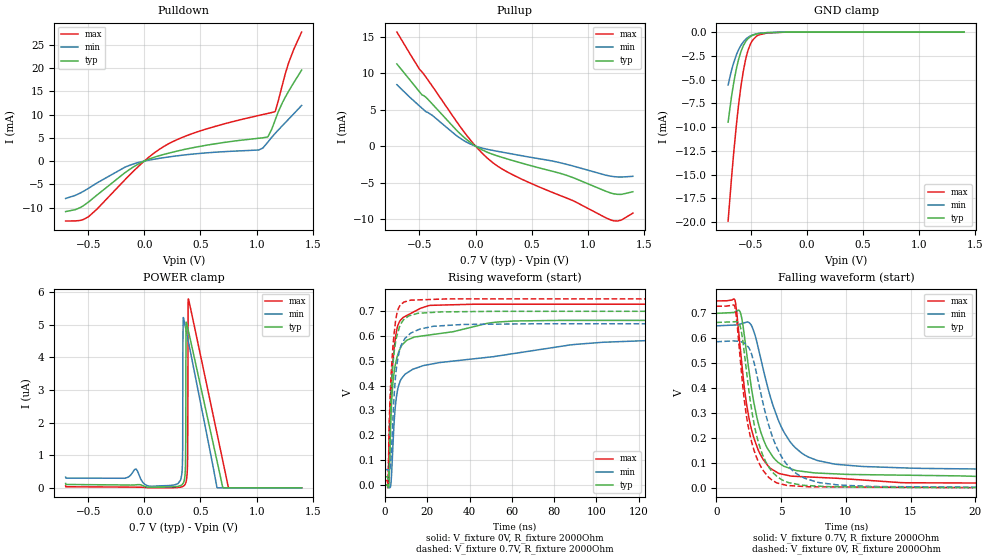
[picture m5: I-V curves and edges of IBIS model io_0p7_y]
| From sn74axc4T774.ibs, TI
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|   io_0p7_y Model
[Model]   io_0p7_y
Model_type   I/O
Polarity   Non-Inverting
Enable   Active-Low
Vinl = 0.21
Vinh = 0.49
Vmeas = 0.35
Vref = 0
Cref = 2pF
Rref = 100000
|   typ   min   max
C_comp   1.852pF   1.651pF   2.136pF
[Model spec]
|subparameter
Vinl   0.21   0.195   0.225
Vinh   0.49   0.455   0.525
| Where Nom  PVT is Nominal Process, 0.7V, 27C
|   Fast PVT is Strong Process,  0.75V, -40C
|   Slow PVT is Weak Process,   0.65V, 130C
[Voltage Range]   0.7   0.65   0.75
|Junction Temperature
[Temperature Range]   27   130   -40
[Pullup Reference]   0.7   0.65   0.75
[Pulldown Reference]   -0   0   0
[Power Clamp Reference]   0.7   0.65   0.75
[GND Clamp Reference]   0   0   0
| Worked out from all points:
|   slope of the pulldown table from 0 to 0.105 V, typ, clamps not added: 111 ohm
|   slope of the pullup table from 0 to 0.105 V, typ, clamps not added: 124 ohm
|   GND clamp passes 1 mA (typ) near -0.54 V on its own axis
|   falling waveform, V_fixture 0.7V, R_fixture 2000Ohm: 20-80 % time 1.59ns typ, 2.42ns min, 1.38ns max; typ from 0.7 V to 0.033 V
|   rising waveform, V_fixture 0V, R_fixture 2000Ohm: 20-80 % time 3.92ns typ, 10.6ns min, 2.96ns max; typ from 0 V to 0.663 V
|   rising waveform, V_fixture 0.7V, R_fixture 2000Ohm: 20-80 % time 2.57ns typ, 3.32ns min, 2.42ns max; typ from 0.033 V to 0.7 V
|   falling waveform, V_fixture 0V, R_fixture 2000Ohm: 20-80 % time 1.39ns typ, 2.07ns min, 1.21ns max; typ from 0.663 V to 0 V
[Pulldown]
|   Voltage   I(typ)   I(min)   I(max)
-700mV    -10.84mA   -8.039mA   -12.88mA
-613.9mV  -10.44mA   -7.366mA   -12.86mA
-496.3mV  -8.79mA    -5.848mA   -11.95mA
-86.8mV   -1.114mA   -543.1uA   -1.949mA
74.9mV    709.2uA    349.2uA    1.494mA
230.3mV   1.783mA    928.3uA    3.893mA
528.5mV   3.299mA    1.714mA    6.718mA
1.018V    4.901mA    2.379mA    9.794mA
1.098V    5.18mA     4.003mA    10.23mA
1.163V    8.678mA    5.897mA    10.62mA
1.282V    14.92mA    8.955mA    20.95mA
1.4V      19.54mA    11.95mA    27.72mA
[GND Clamp]
|   Voltage   I(typ)   I(min)   I(max)
-700mV    -9.473mA   -5.569mA   -19.87mA
-674.8mV  -7.198mA   -4.264mA   -16.07mA
-649.6mV  -5.285mA   -3.192mA   -12.61mA
-622.3mV  -3.629mA   -2.276mA   -9.304mA
-584.5mV  -2.013mA   -1.371mA   -5.599mA
-544.6mV  -1.015mA   -772.1uA   -2.899mA
-521.5mV  -677.6uA   -547uA     -1.878mA
-481.6mV  -348uA     -300.8uA   -843.7uA
-443.8mV  -200.2uA   -174.6uA   -401uA
-351.4mV  -69.33uA   -55.44uA   -97.88uA
-175mV    -6.308uA   -6.304uA   -6.326uA
1.4V      0A         0A         0A
[Pullup]
|   Voltage   I(typ)   I(min)   I(max)
-700mV    11.25mA    8.412mA    15.63mA
-500.5mV  7.467mA    5.518mA    10.57mA
-424.9mV  6.427mA    4.607mA    9.085mA
-145.6mV  1.818mA    1.166mA    2.856mA
-7mV      68.33uA    37.43uA    122.1uA
148.4mV   -1.105mA   -579uA     -2.212mA
263.9mV   -1.677mA   -908.2uA   -3.386mA
410.9mV   -2.34mA    -1.323mA   -4.536mA
793.1mV   -3.921mA   -2.435mA   -7.018mA
1.203V    -6.426mA   -4.123mA   -10.12mA
1.291V    -6.618mA   -4.243mA   -10.17mA
1.4V      -6.259mA   -4.143mA   -9.188mA
[POWER Clamp]
|   Voltage   I(typ)   I(min)   I(max)
-700mV    133.1nA    328.5nA    61.75nA
301.7mV   46.57nA    137.1nA    11.38nA
337.4mV   102.3nA    571.4nA    34.33nA
341.6mV   118.7nA    1.205uA    40.17nA
345.8mV   140.3nA    5.138uA    47.42nA
362.6mV   405.2nA    4.989uA    104.1nA
368.9mV   1.505uA    4.883uA    151.5nA
371mV     4.89uA     4.848uA    174.5nA
385.7mV   4.915uA    4.597uA    910.4nA
392mV     4.819uA    4.489uA    5.793uA
751.1mV   0A         0A         0A
1.4V      0A         0A         0A
[Ramp]
R_load = 2000
|   typ   min   max
dV/dt_r   0.398078/3.88391e-09   0.351677/1.04111e-08   0.437151/2.93764e-09
dV/dt_f   0.400332/1.59305e-09   0.352882/2.41142e-09   0.439509/1.3705e-09
[Falling Waveform]
V_fixture = 0.7V
V_fixture_min = 0.65V
V_fixture_max = 0.75V
R_fixture = 2000Ohm
C_fixture = 0F
|   Time   V(typ)   V(min)   V(max)
0s        700mV      650mV      750mV
1.435ns   705.8mV    653.3mV    753.6mV
1.852ns   704.2mV    657.3mV    560.5mV
2.701ns   404.1mV    652.3mV    237.4mV
3.326ns   242.6mV    542mV      141.6mV
4.074ns   148.1mV    383mV      83.34mV
5.226ns   86.52mV    223.4mV    53.29mV
6.869ns   64.66mV    130.4mV    44.29mV
14.26ns   50.99mV    80.43mV    20.93mV
500ns     32.77mV    61.84mV    17.48mV
[Rising Waveform]
V_fixture = 0V
V_fixture_min = 0V
V_fixture_max = 0V
R_fixture = 2000Ohm
C_fixture = 0F
|   Time   V(typ)   V(min)   V(max)
0s        382.6nV    4.781uV    130.3nV
1.423ns   -8.803mV   -747uV     -3.094mV
1.913ns   10.2mV     -8.954mV   186.6mV
2.666ns   241.7mV    -3.545mV   361.6mV
3.797ns   417.7mV    171.4mV    502.8mV
5.733ns   517.5mV    373.6mV    633.3mV
9.44ns    576mV      446.1mV    679.1mV
20.81ns   604.2mV    485.2mV    723.1mV
124.2ns   663.2mV    581.7mV    728.5mV
500ns     663.5mV    586.1mV    728.6mV
[Rising Waveform]
V_fixture = 0.7V
V_fixture_min = 0.65V
V_fixture_max = 0.75V
R_fixture = 2000Ohm
C_fixture = 0F
|   Time   V(typ)   V(min)   V(max)
0s        32.77mV    61.84mV    17.48mV
1.423ns   24.36mV    60.74mV    17.67mV
1.793ns   37.58mV    54.73mV    168.5mV
2.284ns   177.9mV    65.74mV    333.8mV
3.229ns   425.5mV    174.7mV    495.5mV
4.916ns   571.2mV    432.7mV    656.8mV
7.364ns   646.7mV    556.2mV    725.9mV
12ns      683.3mV    610.7mV    744.7mV
70.67ns   699.9mV    649.6mV    749.9mV
500ns     700mV      650mV      750mV
[Falling Waveform]
|Gnd
V_fixture = 0V
V_fixture_min = 0V
V_fixture_max = 0V
R_fixture = 2000Ohm
C_fixture = 0F
|   Time   V(typ)   V(min)   V(max)
0s        663.5mV    586.1mV    728.6mV
1.435ns   666.5mV    589.2mV    726.1mV
1.913ns   633.9mV    586.2mV    480mV
2.33ns    467.9mV    572.8mV    287.5mV
2.782ns   295.2mV    525.8mV    173.3mV
3.342ns   167.7mV    402.3mV    94.66mV
4.057ns   83.08mV    249.4mV    41.77mV
5.042ns   33.1mV     124.5mV    14.98mV
7.183ns   8.87mV     32.65mV    4.218mV
500ns     374.6nV    4.907uV    113.5nV
